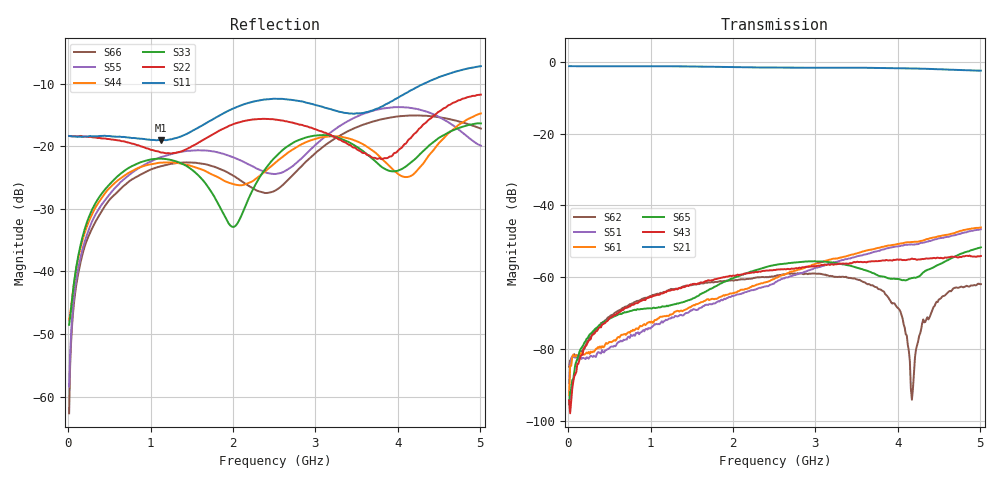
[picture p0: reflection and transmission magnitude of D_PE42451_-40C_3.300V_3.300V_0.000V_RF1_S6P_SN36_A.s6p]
! Device ID: PE42451
! Serial: 36
! Insertion: A
! Temp: -40C
! VDD: 3.300
! Control_Hi: 100.000
! Control_Lo: 0.000
! Logic State: RF1
! Port 1: RFC
! Port 2: RF1
! Port 3: RF2
! Port 4: RF3
! Port 5: RF4
! Port 6: RF5
! V1 = 3.30
! V2 = 0.00
! V3 = 0.00
! V4 = 0.00
! IDD: 1.609800e-05
#  Hz  S  RI  R  50
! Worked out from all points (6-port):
!   401 points, 10 MHz to 5.01 GHz, reference 50 ohm
!   strongest paths, dB at 10 MHz, 1.26 GHz, 2.51 GHz, 3.76 GHz, 5.01 GHz:
!     S21: -1.2, -1.3, -1.6, -1.7, -2.5
!     S43: -94.3, -63.4, -58.0, -55.5, -54.1
!     S65: -95.3, -67.7, -56.6, -59.5, -51.6
!     S61: -92.7, -70.2, -60.3, -51.8, -46.1
!     S51: -89.4, -71.1, -61.5, -52.7, -46.6
!     S62: -84.9, -63.3, -59.6, -63.2, -61.9
!   lowest |S11| = -19.0 dB at 1.123 GHz (marker M1), VSWR 1.25, Z = 57.1 - j9.7 ohm
!   |S11| at or under -10 dB: start of sweep to 4.314 GHz
